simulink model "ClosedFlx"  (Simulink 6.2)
settings: Solver=ode113  StartTime=0.0  StopTime=40  MaxStep=0.001  RelTol=1e-3
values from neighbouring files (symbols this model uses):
  Kp = om^2*Iy/(l*T)    (= 0.554556771732)    [run.m]    (also in run3.m = 0.554540604935)
  Kr = 2*0.85*om*Iy/(l*T)    (= 1.03530256089)    [run.m]    (also in run3.m = 1.03527237908)
  r2d = 180/pi    (= 57.2957795131)    [Pl.m]    (also in Plc.m; run.m; run2.m; run3.m)
  wd = 7    [run.m]    (also in run3.m)
  wd2 = 16    [run.m]    (also in run3.m)
  wf = 9    [run.m]    (also in run3.m)
  wn = 7.4    [run.m]    (also in run3.m)
  wn2 = 16.8    [run.m]    (also in run3.m)
  zd = 0.2    [run.m]    (also in run3.m)
  zd2 = 0.2    [run.m]    (also in run3.m)
  zn = 0.02    [run.m]    (also in run3.m)
  zn2 = 0.015    [run.m]    (also in run3.m)
undefined symbols (not defined in the file or in its folder): Av, Bv, Cv, Dv

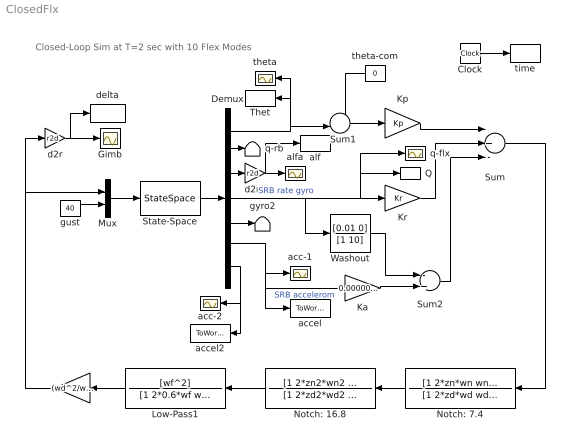
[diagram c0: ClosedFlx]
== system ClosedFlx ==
  note: Closed-Loop Sim at T=2 sec with 10 Flex Modes
  " " : Gain  Orientation=left  Gain=(wd^2/wn^2)*(wd2^2/wn2^2)
  Clock : Clock
  Demux : Demux  Outputs=7
  Gimb : Scope
  Ka : Gain  Gain=0.0000015
  Kp : Gain  Gain=Kp
  Kr : Gain  Gain=Kr
  Low-Pass1 : TransferFcn  Orientation=left  Numerator=[wf^2]  Denominator=[1 2*0.6*wf wf^2]
  Mux : Mux  Inputs=2
  Notch: 16.8 : TransferFcn  Orientation=left  Numerator=[1 2*zn2*wn2 wn2^2]  Denominator=[1 2*zd2*wd2 wd2^2]
  Notch: 7.4 : TransferFcn  Orientation=left  Numerator=[1 2*zn*wn wn^2]  Denominator=[1 2*zd*wd wd^2]
  Q : ToWorkspace  VariableName=q  SampleTime=-1  SaveFormat=Array
  State-Space : StateSpace  A=Av  B=Bv  C=Cv  D=Dv
  Sum : Sum  Inputs=-+-
  Sum1 : Sum  Inputs=+-|
  Sum2 : Sum  Inputs=-+
  Thet : ToWorkspace  VariableName=theta  SampleTime=-1  SaveFormat=Array
  Washout : TransferFcn  Numerator=[0.01 0]  Denominator=[1 10]
  acc-1 : Scope
  acc-2 : Scope
  accel : ToWorkspace  VariableName=accel_1  SampleTime=-1  SaveFormat=Array
  accel2 : ToWorkspace  VariableName=accel_2  SampleTime=-1  SaveFormat=Array
  alf : ToWorkspace  VariableName=alpha  SampleTime=-1  SaveFormat=Array
  alfa : Scope
  d2r : Gain  Gain=r2d
  d2r1 : Gain  Gain=r2d
  delta : ToWorkspace  VariableName=delta  SampleTime=-1  SaveFormat=Array
  gust : Constant  Value=40
  gyro2 : Terminator
  q-flx : Scope
  q-rb : Terminator
  theta : Scope
  theta-com : Constant  Orientation=left  Value=0
  time : ToWorkspace  VariableName=time  SampleTime=-1  SaveFormat=Array
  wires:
  Mux/1 -> State-Space/1
  gust/1 -> Mux/2
  theta-com/1 -> Sum1/1
  Notch: 16.8/1 -> Low-Pass1/1
  Kr/1 -> Sum/2
  Kp/1 -> Sum/1
  Sum1/1 -> Kp/1
  Sum/1 -> Notch: 7.4/1
  Clock/1 -> time/1
  Demux/1 -> Thet/1, theta/1, Sum1/2
  Demux/2 -> q-rb/1
  Demux/4 -> Kr/1, Q/1, q-flx/1, Washout/1  "SRB rate gyro"
  Demux/6 -> Ka/1, accel/1, acc-1/1  "SRB accelerom"
  Demux/7 -> acc-2/1, accel2/1
  State-Space/1 -> Demux/1
  Demux/5 -> gyro2/1
  Ka/1 -> Sum2/2
  Washout/1 -> Sum2/1
  Sum2/1 -> Sum/3
  d2r/1 -> Gimb/1, delta/1
  Demux/3 -> d2r1/1
  d2r1/1 -> alfa/1, alf/1
  " "/1 -> Mux/1, d2r/1
  Low-Pass1/1 -> " "/1
  Notch: 7.4/1 -> Notch: 16.8/1
